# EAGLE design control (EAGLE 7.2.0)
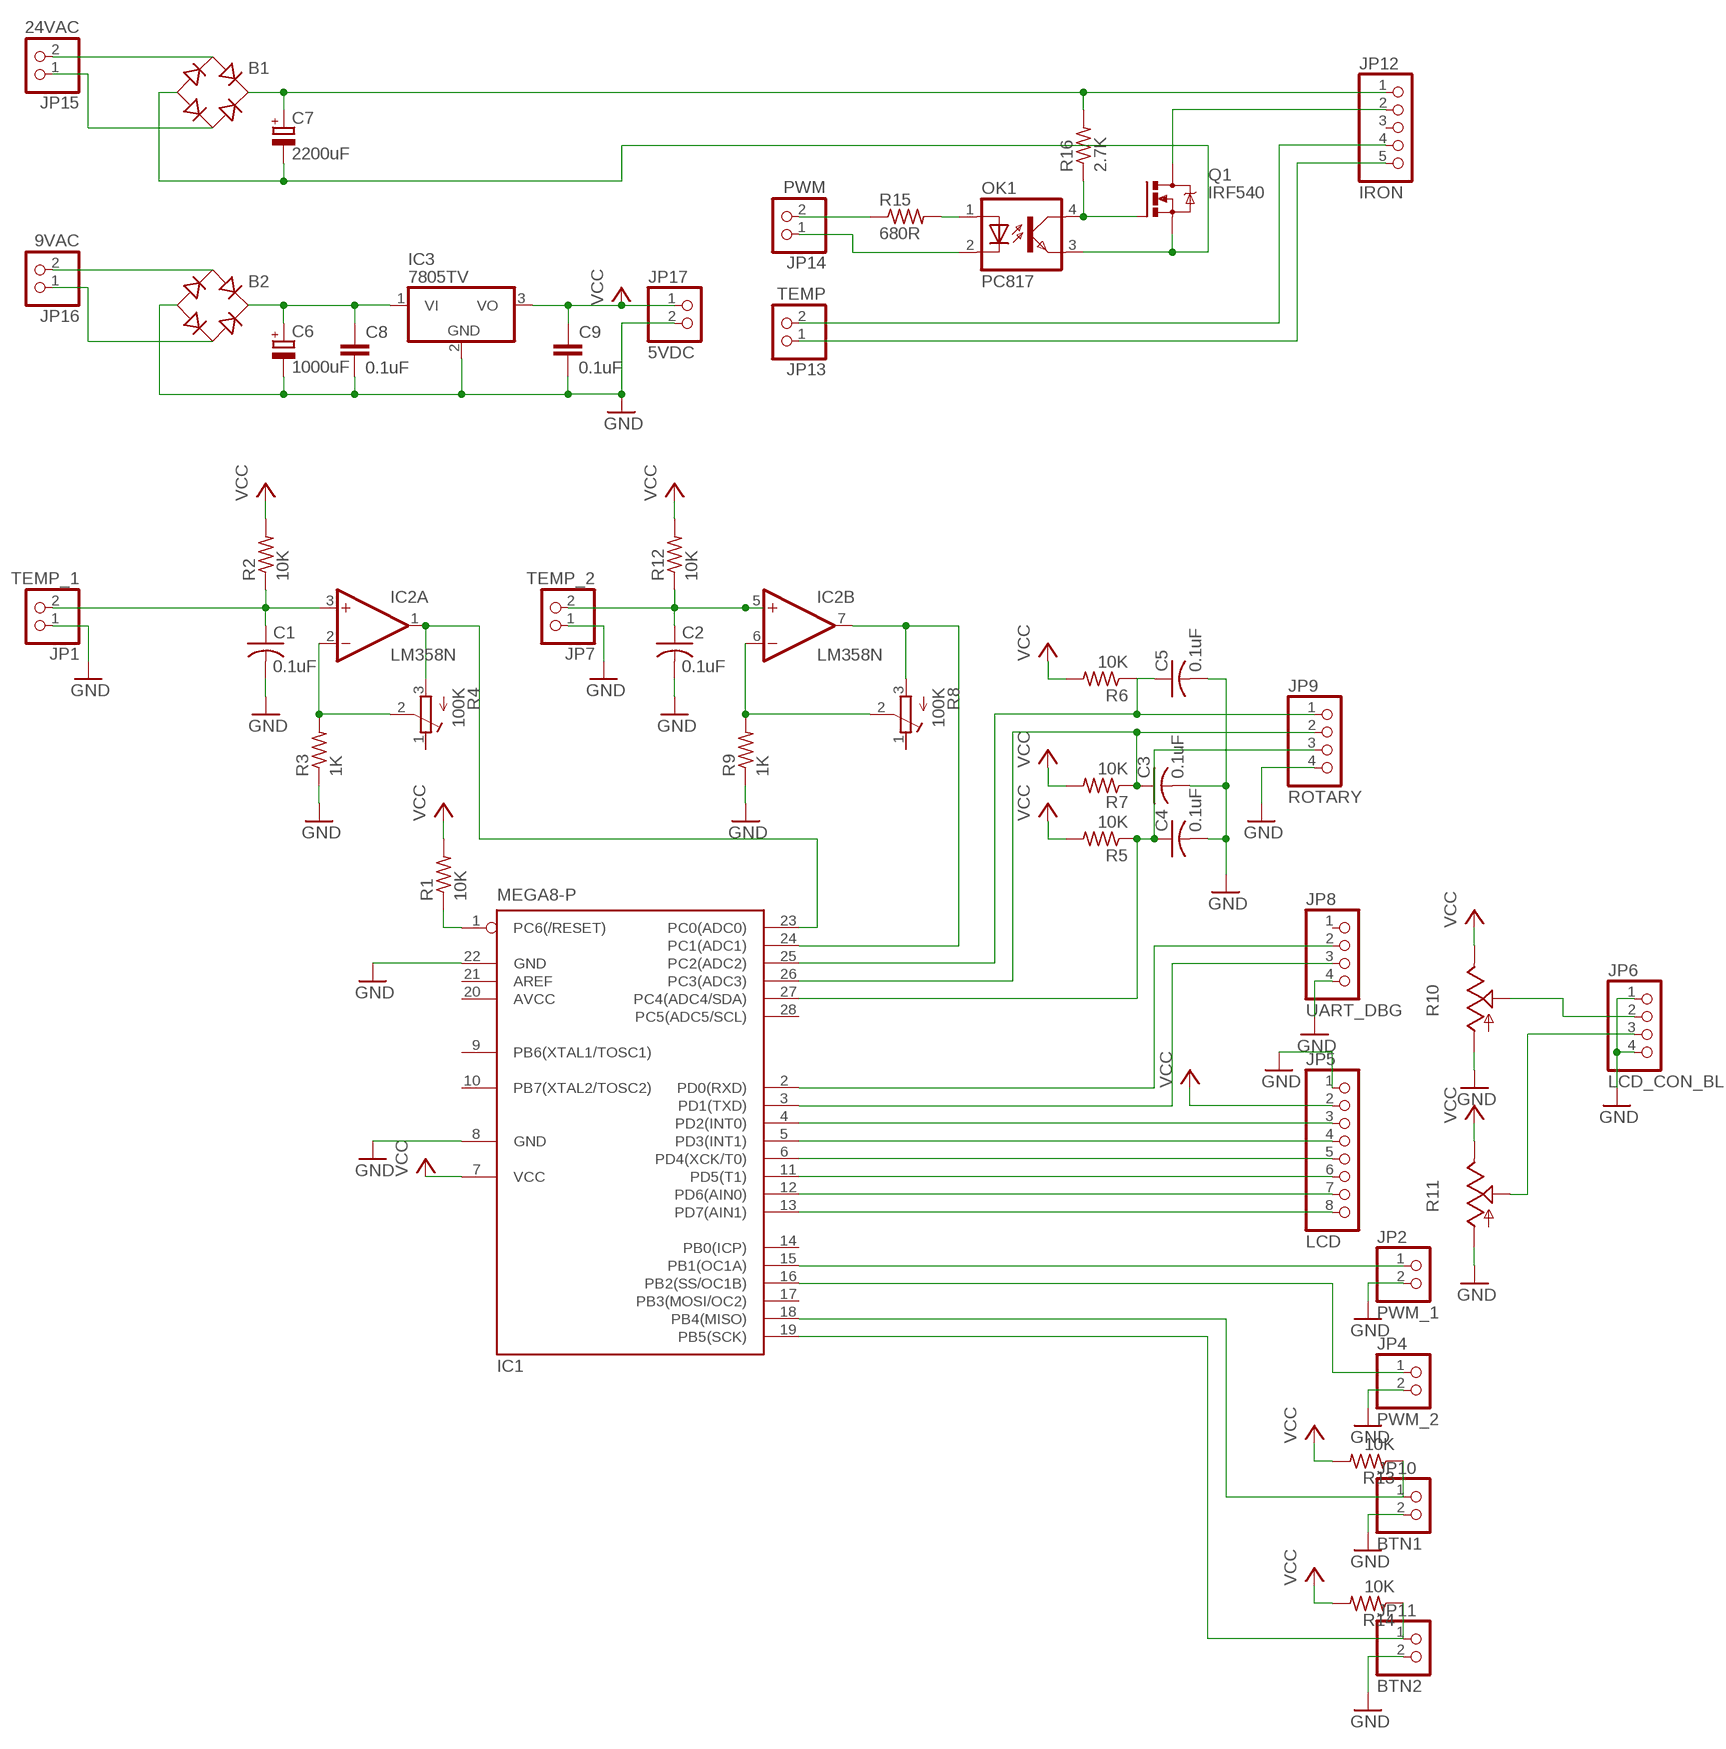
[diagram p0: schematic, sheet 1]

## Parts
B1  RB1A  [RB1A]
B2  RB1A  [RB1A]
C1  0.1uF  C-US025-025X050  [C025-025X050]
C2  0.1uF  C-US025-025X050  [C025-025X050]
C3  0.1uF  C-US025-025X050  [C025-025X050]
C4  0.1uF  C-US025-025X050  [C025-025X050]
C5  0.1uF  C-US025-025X050  [C025-025X050]
C6  1000uF  CPOL-EUE5-8.5  [E5-8,5]
C7  2200uF  CPOL-EUE7.5-18  [E7,5-18]
C8  0.1uF  C-EU050-030X075  [C050-030X075]
C9  0.1uF  C-EU050-030X075  [C050-030X075]
IC1  MEGA8-P  [DIL28-3]
IC2  LM358N  [DIL08]
IC3  7805TV  [TO220V]
JP1  TEMP_1  PINHD-1X2  [1X02]
JP2  PWM_1  PINHD-1X2  [1X02]
JP4  PWM_2  PINHD-1X2  [1X02]
JP5  LCD  PINHD-1X8  [1X08]
JP6  LCD_CON_BL  PINHD-1X4  [1X04]
JP7  TEMP_2  PINHD-1X2  [1X02]
JP8  UART_DBG  PINHD-1X4  [1X04]
JP9  ROTARY  PINHD-1X4  [1X04]
JP10  BTN1  PINHD-1X2  [1X02]
JP11  BTN2  PINHD-1X2  [1X02]
JP12  IRON  PINHD-1X5  [1X05]
JP13  TEMP  PINHD-1X2  [1X02]
JP14  PWM  PINHD-1X2  [1X02]
JP15  24VAC  PINHD-1X2  [1X02]
JP16  9VAC  PINHD-1X2  [1X02]
JP17  5VDC  PINHD-1X2  [1X02]
OK1  PC817  [DIL04]
Q1  IRF540  [TO220BV]
R1  10K  R-US_0207/10  [0207/10]
R2  10K  R-US_0207/10  [0207/10]
R3  1K  R-US_0207/10  [0207/10]
R4  100K  R-TRIMMT93YA  [RTRIMT93YA]
R5  10K  R-US_0207/10  [0207/10]
R6  10K  R-US_0207/10  [0207/10]
R7  10K  R-US_0207/10  [0207/10]
R8  100K  R-TRIMMT93YA  [RTRIMT93YA]
R9  1K  R-US_0207/10  [0207/10]
R10  TRIM_US-B25P  [B25P]
R11  TRIM_US-B25P  [B25P]
R12  10K  R-US_0207/10  [0207/10]
R13  10K  R-US_0207/10  [0207/10]
R14  10K  R-US_0207/10  [0207/10]
R15  680R  R-US_0207/10  [0207/10]
R16  2.7K  R-US_0207/10  [0207/10]

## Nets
GND: B2.- C1.2 C2.2 C3.2 C4.2 C5.2 C6.- C8.2 C9.2 IC1.8(GND) IC1.22(GND) IC3.2(GND) JP1.1 JP2.2 JP4.2 JP5.1 JP6.1 JP6.4 JP7.1 JP8.4 JP9.4 JP10.2 JP11.2 JP17.2 R3.1 R9.1 R10.A R11.A
N$1: IC1.15(PB1(OC1A)) JP2.1
N$2: IC1.1(PC6(/RESET)) R1.1
N$3: C1.1 IC2.3(A:+IN) JP1.2 R2.1
N$4: IC1.23(PC0(ADC0)) IC2.1(A:OUT) R4.3(A)
N$5: IC2.2(A:-IN) R3.2 R4.2(S)
N$6: C4.1 IC1.27(PC4(ADC4/SDA)) JP9.3 R5.1
N$7: C5.1 IC1.25(PC2(ADC2)) JP9.1 R6.1
N$8: C3.1 IC1.26(PC3(ADC3)) JP9.2 R7.1
N$9: IC1.16(PB2(SS/OC1B)) JP4.1
N$10: IC1.24(PC1(ADC1)) IC2.7(B:OUT) R8.3(A)
N$11: IC2.6(B:-IN) R8.2(S) R9.2
N$12: IC1.13(PD7(AIN1)) JP5.8
N$13: IC1.12(PD6(AIN0)) JP5.7
N$14: IC1.11(PD5(T1)) JP5.6
N$15: IC1.6(PD4(XCK/T0)) JP5.5
N$16: IC1.5(PD3(INT1)) JP5.4
N$17: IC1.4(PD2(INT0)) JP5.3
N$18: JP6.2 R10.S
N$19: JP6.3 R11.S
N$20: C2.1 IC2.5(B:+IN) JP7.2 R12.1
N$21: IC1.2(PD0(RXD)) JP8.2
N$22: IC1.3(PD1(TXD)) JP8.3
N$23: IC1.18(PB4(MISO)) JP10.1 R13.1
N$24: IC1.19(PB5(SCK)) JP11.1 R14.1
N$25: B1.AC1 JP15.2
N$26: B1.AC2 JP15.1
N$27: B2.AC1 JP16.2
N$28: B2.AC2 JP16.1
N$31: B2.+ C6.+ C8.1 IC3.1(VI)
N$32: B1.+ C7.+ JP12.1 R16.2
N$33: JP12.2 Q1.D
N$34: OK1.4(COL) Q1.G R16.1
N$35: B1.- C7.- OK1.3(EMIT) Q1.S
N$36: JP12.4 JP13.2
N$37: JP12.5 JP13.1
N$38: JP14.2 R15.1
N$39: OK1.1(A) R15.2
N$40: JP14.1 OK1.2(C)
VCC: C9.1 IC1.7(VCC) IC3.3(VO) JP5.2 JP17.1 R1.2 R2.2 R5.2 R6.2 R7.2 R10.E R11.E R12.2 R13.2 R14.2
Unconnected: IC1.9(PB6(XTAL1/TOSC1)) IC1.10(PB7(XTAL2/TOSC2)) IC1.14(PB0(ICP)) IC1.17(PB3(MOSI/OC2)) IC1.21(AREF) IC1.28(PC5(ADC5/SCL)) JP8.1 JP12.3 R4.1(E) R8.1(E)

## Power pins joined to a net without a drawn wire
AVCC: IC1.20(AVCC)
V-: IC2.4(P:V-)
VCC: IC2.8(P:V+)

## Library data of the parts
B1 B2 = rectifier:RB1A: RECTIFIER 1 A
C1-C5 = rcl:C-US: CAPACITOR, American symbol
C6 C7 = rcl:CPOL-EU: POLARIZED CAPACITOR, European symbol
C8 C9 = rcl:C-EU: CAPACITOR, European symbol
IC1 = atmel:MEGA8-P: MICROCONTROLLER 8 Kbytes FLASH, 1 kbytes SRAM, 512 bytes EEPROM, USART, 4-channel 10 bit ADC, 2-channel 8 bit ADC Pin compatible with Atmega48, ATMega88, ATMega168 Source: avr.lbr; OC_FARNELL: unknown; OC_NEWARK: unknown
IC2 = linear:LM358: OP AMP also LM158; LM258; LM2904 Source: http://cache.national.com/ds/LM/LM158.pdf
IC3 = linear:78*: Positive VOLTAGE REGULATOR Source: http://cache.national.com/ds/LM/LM78L05.pdf http://www.fairchildsemi.com/ds/LM/LM7805.pdf
JP1 JP2 JP4 JP7 JP10 JP11 JP13-JP17 = pinhead:PINHD-1X2: PIN HEADER
JP5 = pinhead:PINHD-1X8: PIN HEADER
JP6 JP8 JP9 = pinhead:PINHD-1X4: PIN HEADER
JP12 = pinhead:PINHD-1X5: PIN HEADER
OK1 = optocoupler:PC817: SHARP OPTO COUPLER; MPN: PC817X4J000F; OC_FARNELL: 9707727; OC_NEWARK: 97K7059
Q1 = transistor-power:IRF540: HEXFET Power MOSFET
R1-R3 R5-R7 R9 R12-R16 = rcl:R-US_: RESISTOR, American symbol
R4 R8 = rcl:R-TRIMM: Trimm resistor
R10 R11 = pot:TRIM_US-: POTENTIOMETER

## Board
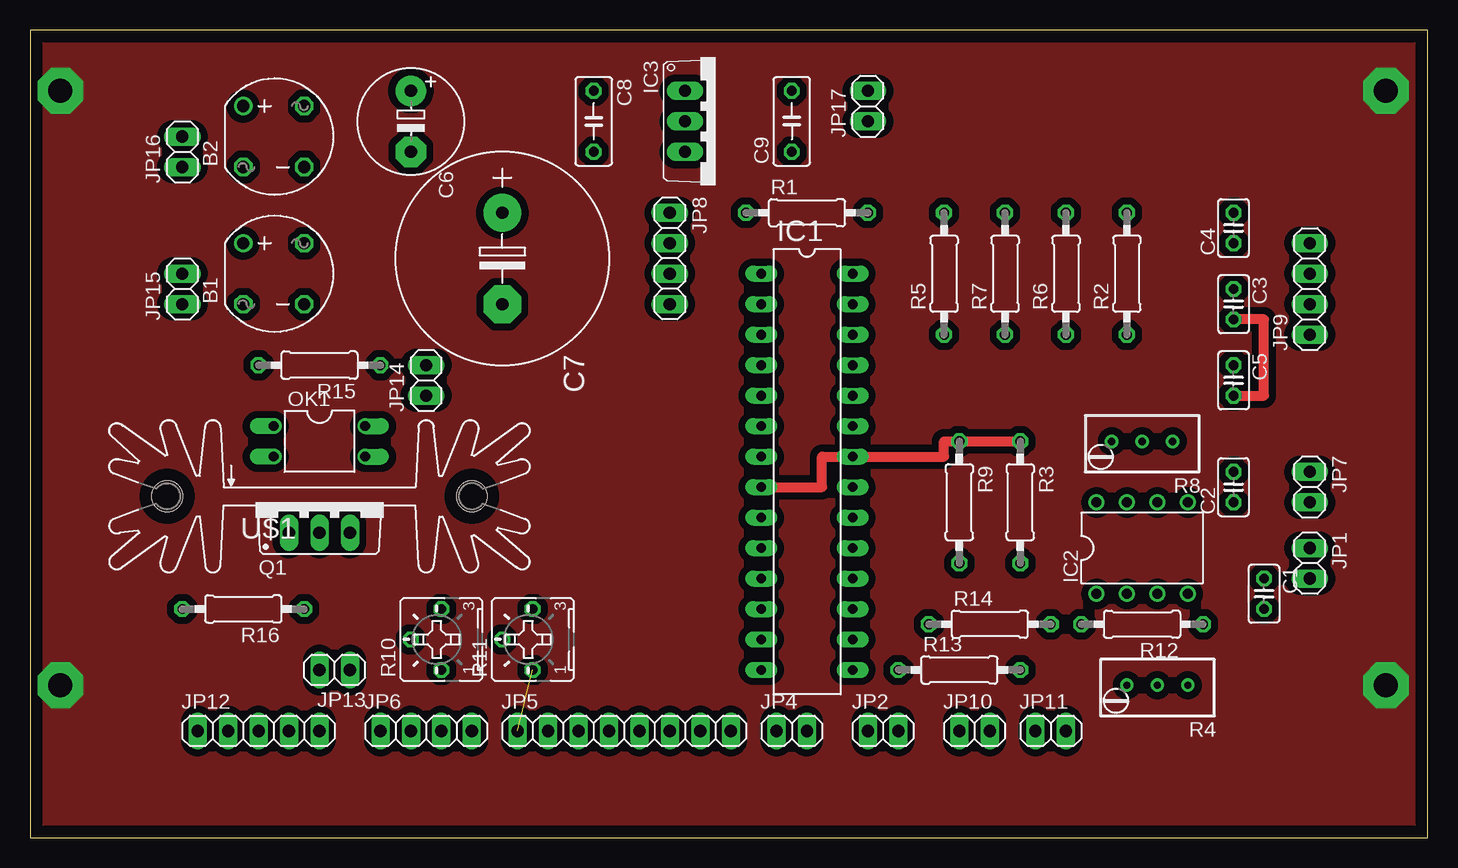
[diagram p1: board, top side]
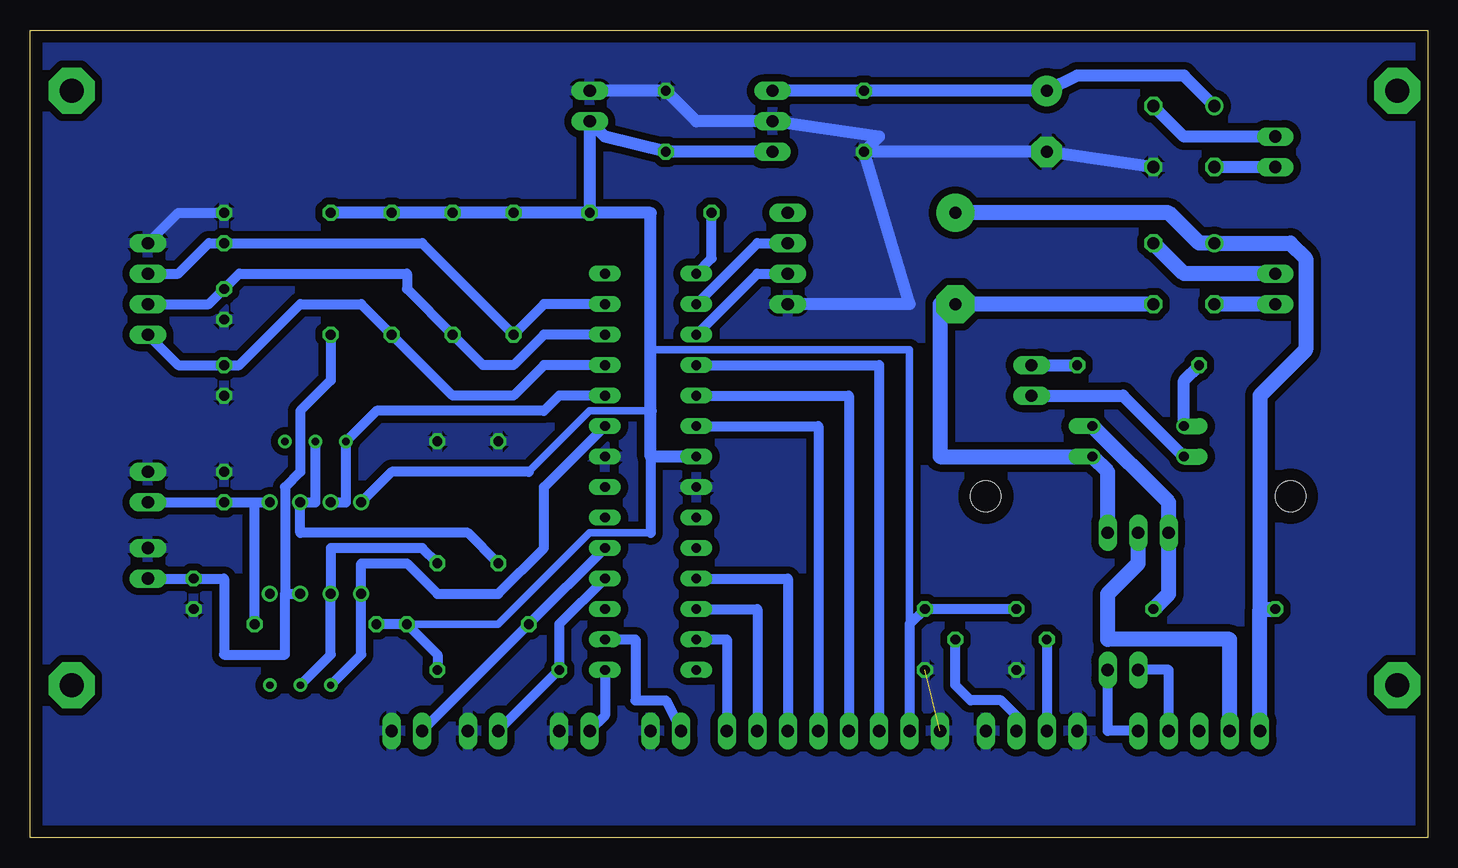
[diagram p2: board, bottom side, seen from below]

Size 116.51 x 67.3 mm. Coordinates in mm from the lower left corner, seen from the top.
Outline: 0,0 116.51,0 116.51,67.3 0,67.3 0,0
Copper layers (1*16): Top 0.035mm / dielectric 1.5mm / Bottom 0.035mm
Design rules "default *": minimum track width 10mil, minimum drill 24mil, track to track 24mil, track to pad 24mil, pad to pad 24mil, via to via 24mil, smd to smd 24mil, copper to edge 40mil, drill to drill 8mil, minimum pad ring 10mil, minimum via ring 8mil, stop-mask expansion 4mil, vias tented up to drill 0mil, thermal gap 10mil

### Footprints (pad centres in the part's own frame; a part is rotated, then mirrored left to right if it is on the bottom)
RB1A = drill 1.016: + -2.54,2.54 | drill 1.016 octagon: - 2.54,-2.54; AC1 2.54,2.54; AC2 -2.54,-2.54
C025-025X050 = drill 0.813 octagon: 1 -1.27,0; 2 1.27,0
E5-8,5 = drill 1.016 pad 2.54: + -2.54,0 | drill 1.016 pad 2.54 octagon: - 2.54,0
E7,5-18 = drill 1.016 pad 3.15: + -3.81,0 | drill 1.016 pad 3.15 octagon: - 3.81,0
C050-030X075 = drill 0.813 octagon: 1 -2.54,0; 2 2.54,0
DIL28-3 = drill 0.813 long: 1 -16.51,-3.81; 2 -13.97,-3.81; 3 -11.43,-3.81; 4 -8.89,-3.81; 5 -6.35,-3.81; 6 -3.81,-3.81; 7 -1.27,-3.81; 8 1.27,-3.81; 9 3.81,-3.81; 10 6.35,-3.81; 11 8.89,-3.81; 12 11.43,-3.81; 13 13.97,-3.81; 14 16.51,-3.81; 15 16.51,3.81; 16 13.97,3.81; 17 11.43,3.81; 18 8.89,3.81; 19 6.35,3.81; 20 3.81,3.81; 21 1.27,3.81; 22 -1.27,3.81; 23 -3.81,3.81; 24 -6.35,3.81; 25 -8.89,3.81; 26 -11.43,3.81; 27 -13.97,3.81; 28 -16.51,3.81
DIL08 = drill 0.813 pad 1.27: 1 -3.81,-3.81; 2 -1.27,-3.81; 3 1.27,-3.81; 4 3.81,-3.81; 5 3.81,3.81; 6 1.27,3.81; 7 -1.27,3.81; 8 -3.81,3.81
TO220V = drill 1.016 long: 1 -2.54,-2.54; 2 0,-2.54; 3 2.54,-2.54
1X02 = drill 1.016 long: 1 -1.27,0; 2 1.27,0
1X08 = drill 1.016 long: 1 -8.89,0; 2 -6.35,0; 3 -3.81,0; 4 -1.27,0; 5 1.27,0; 6 3.81,0; 7 6.35,0; 8 8.89,0
1X04 = drill 1.016 long: 1 -3.81,0; 2 -1.27,0; 3 1.27,0; 4 3.81,0
1X05 = drill 1.016 long: 1 -5.08,0; 2 -2.54,0; 3 0,0; 4 2.54,0; 5 5.08,0
DIL04 = drill 0.813 offset: 1 -1.27,-3.81; 2 1.27,-3.81; 3 1.27,3.81; 4 -1.27,3.81
TO220BV = drill 1.016 long: D 0,-2.54; G -2.54,-2.54; S 2.54,-2.54
0207/10 = drill 0.813 octagon: 1 -5.08,0; 2 5.08,0
RTRIMT93YA = drill 0.61: 1 0,-2.54; 2 0,0; 3 0,2.54
B25P = drill 0.813 octagon: A -2.54,0; E 2.54,0; S 0,2.54
SK104 = hole 2.54: -12.7,-0.762; 12.7,-0.762

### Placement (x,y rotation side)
B1  20.32,46.99 0 top
B2  20.32,58.42 0 top
C1  102.87,20.32 270 top
C2  100.33,29.21 90 top
C3  100.33,44.45 270 top
C4  100.33,50.8 90 top
C5  100.33,38.1 270 top
C6  31.75,59.69 270 top
C7  39.37,48.26 270 top
C8  46.99,59.69 270 top
C9  63.5,59.69 90 top
IC1  64.77,30.48 270 top
IC2  92.71,24.13 0 top
IC3  57.15,59.69 270 top
JP1  106.68,22.86 270 top
JP2  71.12,8.89 0 top
JP4  63.5,8.89 0 top
JP5  49.53,8.89 0 top
JP6  33.02,8.89 0 top
JP7  106.68,29.21 270 top
JP8  53.34,48.26 270 top
JP9  106.68,45.72 90 top
JP10  78.74,8.89 0 top
JP11  85.09,8.89 0 top
JP12  19.05,8.89 0 top
JP13  25.4,13.97 180 top
JP14  33.02,38.1 90 top
JP15  12.7,45.72 90 top
JP16  12.7,57.15 90 top
JP17  69.85,60.96 90 top
OK1  24.13,33.02 270 top
Q1  24.13,27.94 0 top
R1  64.77,52.07 0 top
R2  91.44,46.99 90 top
R3  82.55,27.94 270 top
R4  93.98,12.7 90 top
R5  76.2,46.99 90 top
R6  86.36,46.99 90 top
R7  81.28,46.99 90 top
R8  92.71,33.02 90 top
R9  77.47,27.94 270 top
R10  34.29,16.51 90 top
R11  41.91,16.51 90 top
R12  92.71,17.78 180 top
R13  77.47,13.97 0 top
R14  80.01,17.78 0 top
R15  24.13,39.37 180 top
R16  17.78,19.05 180 top
U$1  [SK104]  24.13,29.21 0 top

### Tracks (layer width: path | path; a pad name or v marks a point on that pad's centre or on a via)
GND  (1 unrouted)
  Top 0.813: IC1.8 66.04,29.21 66.04,31.75 IC1.22 76.2,31.75 76.2,33.02 R9.1 R3.1 | C5.2 102.87,36.83 102.87,43.18 C3.2
  Bottom 0.813: JP9.4 104.14,52.07 C4.2
  Bottom 1.016: B2.- C6.- C8.2 | C8.2 45.72,58.42 IC3.2 60.96,59.69 C9.2 JP17.2 | C8.2 43.18,44.45 JP8.4
  pour Bottom: -1.27,68.58 -1.27,1.27 118.11,1.27 118.11,68.58
MNT  (via drill 2 pad 3.81)
  other vias: 2.54,62.23 113.03,12.7 2.54,12.7 113.03,62.23
  pour Top: -1.27,68.58 -1.27,-1.27 118.11,-1.27 118.11,68.58
N$1
  Bottom 0.813: IC1.15 68.58,10.16 JP2.1
N$2
  Bottom 0.813: IC1.1 59.69,48.26 R1.1
N$3
  Bottom 0.813: JP1.2 C1.1 100.33,21.59 100.33,15.24 95.25,15.24 95.25,20.32 | 95.25,20.32 IC2.3 | R2.1 91.44,38.1 93.98,35.56 93.98,30.48 95.25,29.21 95.25,20.32
N$4
  Bottom 0.813: R4.3 88.9,15.24 IC2.1 88.9,22.86 85.09,22.86 82.55,20.32 77.47,20.32 73.66,24.13 73.66,29.21 IC1.23
N$5
  Bottom 0.813: R4.2 91.44,15.24 IC2.2 91.44,24.13 83.82,24.13 R3.2
N$6
  Bottom 0.813: JP9.3 104.14,46.99 101.6,49.53 C4.1 83.82,49.53 R5.1 73.66,44.45 IC1.27
N$7
  Bottom 0.813: JP9.1 104.14,39.37 C5.1 99.06,39.37 93.98,44.45 88.9,44.45 R6.1 81.28,36.83 76.2,36.83 73.66,39.37 IC1.25
N$8
  Bottom 0.813: JP9.2 101.6,44.45 C3.1 99.06,46.99 85.09,46.99 85.09,45.72 R7.1 78.74,39.37 76.2,39.37 73.66,41.91 IC1.26
N$9
  Bottom 0.813: IC1.16 66.04,16.51 66.04,11.43 63.5,11.43 JP4.1
N$10
  Bottom 0.813: IC2.7 90.17,27.94 R8.3 87.63,35.56 73.66,35.56 72.39,36.83 IC1.24
N$11
  Bottom 0.813: R8.2 92.71,27.94 IC2.6 93.98,25.4 80.01,25.4 R9.2
N$12
  Bottom 0.813: IC1.13 58.42,16.51 JP5.8
N$13
  Bottom 0.813: IC1.12 55.88,19.05 JP5.7
N$14
  Bottom 0.813: IC1.11 53.34,21.59 JP5.6
N$15
  Bottom 0.813: IC1.6 50.8,34.29 JP5.5
N$16
  Bottom 0.813: IC1.5 48.26,36.83 JP5.4
N$17
  Bottom 0.813: IC1.4 45.72,39.37 JP5.3
N$18
  Bottom 0.813: R10.S JP6.2
N$19
  Bottom 0.813: JP6.3 34.29,10.16 35.56,11.43 38.1,11.43 39.37,12.7 R11.S
N$20
  Bottom 0.813: JP7.2 C2.1 97.79,27.94 | 97.79,27.94 IC2.5 | R12.1 97.79,27.94
N$21
  Bottom 0.813: IC1.2 55.88,49.53 JP8.2
N$22
  Bottom 0.813: IC1.3 55.88,46.99 JP8.3
N$23
  Bottom 0.813: IC1.18 72.39,17.78 R13.1 JP10.1
N$24
  Bottom 0.813: IC1.19 R14.1 JP11.1
N$25
  Bottom 1.27: JP15.2 20.32,46.99 B1.AC1
N$26
  Bottom 1.27: JP15.1 B1.AC2
N$27
  Bottom 1.016: JP16.2 20.32,58.42 B2.AC1
N$28
  Bottom 1.016: JP16.1 B2.AC2
N$31
  Bottom 1.016: B2.+ 20.32,63.5 29.21,63.5 C6.+ C8.1 IC3.1
N$32
  Bottom 1.27: C7.+ 21.59,52.07 19.05,49.53 B1.+ 11.43,49.53 10.16,48.26 10.16,40.64 13.97,36.83 13.97,19.05 | JP12.1 13.97,19.05 | 13.97,19.05 R16.2
N$33
  Bottom 1.27: JP12.2 16.51,16.51 26.67,16.51 26.67,20.32 24.13,22.86 Q1.D
N$34
  Bottom 1.27: OK1.4 21.59,27.94 Q1.G 21.59,20.32 R16.1
N$35
  Bottom 1.27: B1.- C7.- 40.64,44.45 40.64,31.75 OK1.3 26.67,30.48 Q1.S
N$36
  Bottom 0.813: JP12.4 21.59,13.97 JP13.2
N$37
  Bottom 0.813: JP12.5 26.67,8.89 JP13.1
N$38
  Bottom 1.016: JP14.2 R15.1
N$39
  Bottom 1.016: OK1.1 20.32,38.1 R15.2
N$40
  Bottom 1.016: JP14.1 25.4,36.83 OK1.2
VCC
  Bottom 0.61: 64.77,40.64 43.18,40.64 43.18,17.78 | 64.77,25.4 69.85,25.4 77.47,17.78 R14.2 | 64.77,35.56 69.85,35.56 74.93,30.48
  Bottom 0.813: R10.E R11.E 43.18,17.78 JP5.2 | R13.2 82.55,15.24 R14.2 R12.2 | 64.77,31.75 64.77,25.4 | 74.93,30.48 86.36,30.48 IC2.8
  Bottom 1.016: IC3.3 C9.1 68.58,58.42 JP17.1 R1.2 | R1.2 R5.2 R7.2 R6.2 R2.2 | IC1.7 64.77,31.75 64.77,35.56 64.77,40.64 64.77,52.07 R1.2

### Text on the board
tDocu: SOLDERING STATION | 5VDC | 9VAC | 24VAC | ROTARY | T° | T° | IRON | LCD_CON | LCD DATA | BTN 1-2 | PWM1 | PWM2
